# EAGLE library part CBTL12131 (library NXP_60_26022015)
DisplayPort multiplexer for bidirectional video AAL Eindhoven MK
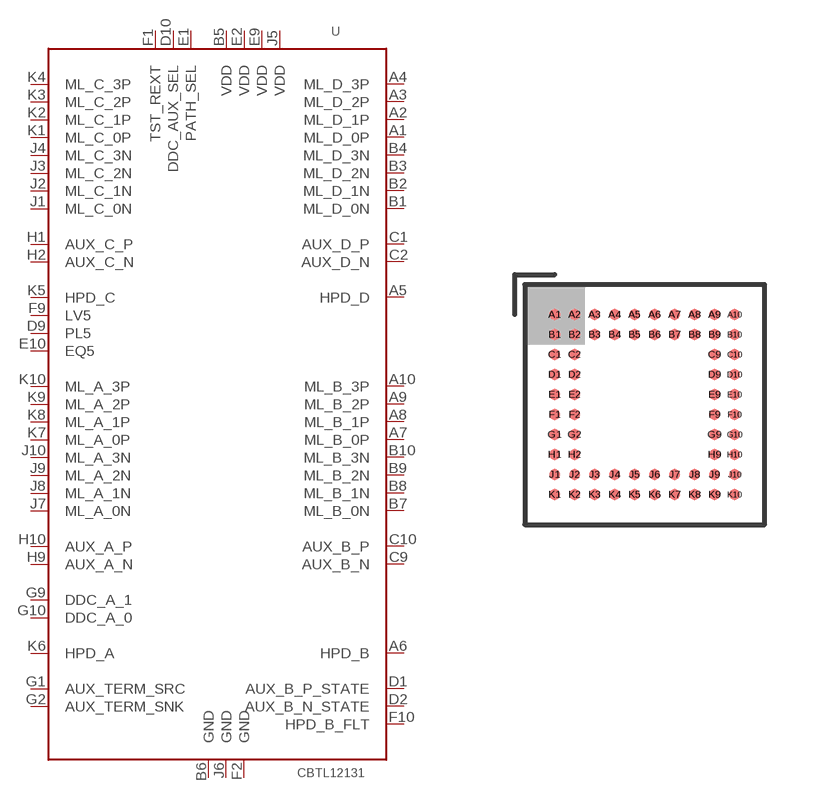
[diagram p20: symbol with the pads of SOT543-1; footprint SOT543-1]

Designator prefix U

## CBTL12131ET  [SOT543-1]
A1  ML_D_0P
A2  ML_D_1P
A3  ML_D_2P
A4  ML_D_3P
A5  HPD_D  in
A6  HPD_B
A7  ML_B_0P
A8  ML_B_1P
A9  ML_B_2P
A10  ML_B_3P
B1  ML_D_0N
B2  ML_D_1N
B3  ML_D_2N
B4  ML_D_3N
B5  VDD  pwr
B6  GND  pwr
B7  ML_B_0N
B8  ML_B_1N
B9  ML_B_2N
B10  ML_B_3N
C1  AUX_D_P
C2  AUX_D_N
C9  AUX_B_N
C10  AUX_B_P
D1  AUX_B_P_STATE  out
D2  AUX_B_N_STATE  out
D9  PL5  in
D10  DDC_AUX_SEL  in
E1  PATH_SEL  in
E2  VDD  pwr
E9  VDD  pwr
E10  EQ5  in
F1  TST_REXT  in
F2  GND  pwr
F9  LV5  in
F10  HPD_B_FLT  out
G1  AUX_TERM_SRC  in
G2  AUX_TERM_SNK  in
G9  DDC_A_1
G10  DDC_A_0
H1  AUX_C_P
H2  AUX_C_N
H9  AUX_A_N
H10  AUX_A_P
J1  ML_C_0N
J2  ML_C_1N
J3  ML_C_2N
J4  ML_C_3N
J5  VDD  pwr
J6  GND  pwr
J7  ML_A_0N
J8  ML_A_1N
J9  ML_A_2N
J10  ML_A_3N
K1  ML_C_0P
K2  ML_C_1P
K3  ML_C_2P
K4  ML_C_3P
K5  HPD_C  out
K6  HPD_A  out
K7  ML_A_0P
K8  ML_A_1P
K9  ML_A_2P
K10  ML_A_3P

## Footprint SOT543-1 (pad centres in mm)
SOT543-1 TFBGA64: plastic thin fine-pitch ball grid array package; 64 balls; body 6 x 6 x 0.8 mm JEDEC: MO195 IEC: --
smd 0.275 x 0.275: A1 -2.25,2.25; A2 -1.75,2.25; A3 -1.25,2.25; A4 -0.75,2.25; A5 -0.25,2.25; A6 0.25,2.25; A7 0.75,2.25; A8 1.25,2.25; A9 1.75,2.25; A10 2.25,2.25; B1 -2.25,1.75; B2 -1.75,1.75; B3 -1.25,1.75; B4 -0.75,1.75; B5 -0.25,1.75; B6 0.25,1.75; B7 0.75,1.75; B8 1.25,1.75; B9 1.75,1.75; B10 2.25,1.75; C1 -2.25,1.25; C2 -1.75,1.25; C9 1.75,1.25; C10 2.25,1.25; D1 -2.25,0.75; D2 -1.75,0.75; D9 1.75,0.75; D10 2.25,0.75; E1 -2.25,0.25; E2 -1.75,0.25; E9 1.75,0.25; E10 2.25,0.25; F1 -2.25,-0.25; F2 -1.75,-0.25; F9 1.75,-0.25; F10 2.25,-0.25; G1 -2.25,-0.75; G2 -1.75,-0.75; G9 1.75,-0.75; G10 2.25,-0.75; H1 -2.25,-1.25; H2 -1.75,-1.25; H9 1.75,-1.25; H10 2.25,-1.25; J1 -2.25,-1.75; J2 -1.75,-1.75; J3 -1.25,-1.75; J4 -0.75,-1.75; J5 -0.25,-1.75; J6 0.25,-1.75; J7 0.75,-1.75; J8 1.25,-1.75; J9 1.75,-1.75; J10 2.25,-1.75; K1 -2.25,-2.25; K2 -1.75,-2.25; K3 -1.25,-2.25; K4 -0.75,-2.25; K5 -0.25,-2.25; K6 0.25,-2.25; K7 0.75,-2.25; K8 1.25,-2.25; K9 1.75,-2.25; K10 2.25,-2.25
